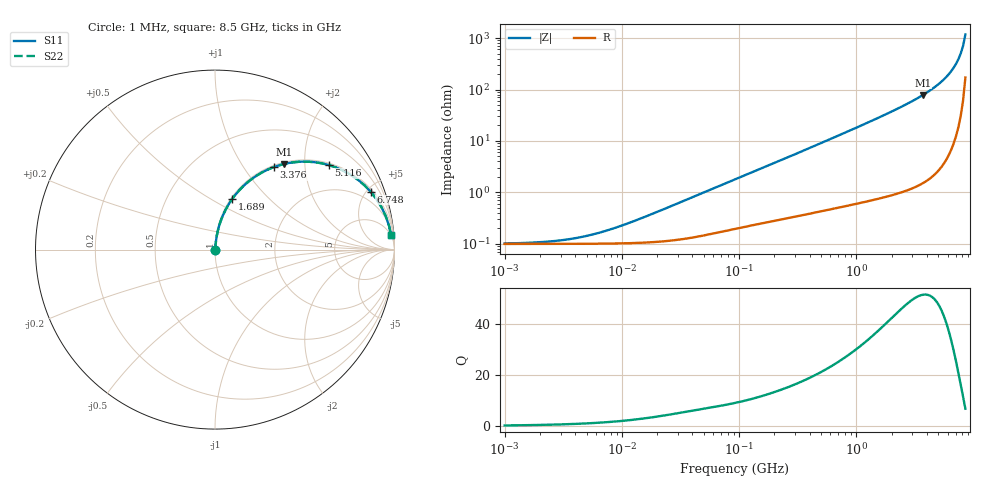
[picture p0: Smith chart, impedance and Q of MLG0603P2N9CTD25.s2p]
! S-Parameter Data Generated by TDK Corporation
! Copyright(C) 2025 TDK Corporation.
! All Rights Reserved.
! TDK P/N: MLG0603P2N9CTD25 (SMD / SMT Inductor (Coil))
! Property: L=2.9nH at 500MHz
! Size(LxWxT): 0.6x0.3x0.3mm
! Model Type: s2p (Touchstone File Format Version 1.0)
! Frequency: DC=Yes Start=1MHz Stop=8500MHz 198points Log-sweep
! Model Generated on Feb. 6, 2025
! Terms and conditions regarding TDK Simulation Models:
! 1)This simulation model is being provided solely for informational
!  purposes. Please refer to the specifications of the products in
!  terms of detailed characteristics of such products.
! 2)In no event shall TDK Corporation of any of its subsidiaries be
!  liable for any loss or damage arising, directly or indirectly,
!  from any information contained in this simulation model, including,
!  but not limited to loss or damages arising from any inaccuracies,
!  omissions or errors in connection with such information.
! 3)Any and all copyrights on this simulation model are owned by
!  TDK Corporation.  Duplication or redistribution of this simulation
!  model without prior written permission from TDK Corporation
!  is prohibited.
! 4)This simulation model is subject to any modification or change
!  without any prior notice.
! 5)Neither TDK Corporation nor any of its subsidiaries shall make any
!  warranty, express or implied, including but not limited to the
!  correctness, implied warranties of merchantability and fitness for
!  a particular purpose with respect to this simulation models.
! 6)The use of this simulation model shall be deemed to have consented
!  to the terms and conditions hereof.
! Port Assignments:
!  1 ---@@@--- 2
! Applicable Conditions:
!  Temperature = 25 degC
!  DC Bias Current = 0 A
!  Small Signal Operation
# Hz S MA R 50
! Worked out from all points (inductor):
!   197 points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, 1 MHz to 8.5 GHz, reference 50 ohm
!   read as one part in series: L = 3.22 nH near 15.95 MHz
!   highest Q = 51.5 at 3.703 GHz (marker M1), where L = 3.37 nH
!   S11 on the Smith chart (normalised r, x): 1 MHz: 1.00, +0.00; 1.689 GHz: 1.02, +0.62; 3.376 GHz: 1.03, +1.39; 5.116 GHz: 1.06, +2.64; 6.748 GHz: 1.18, +5.29; 8.5 GHz: 4, +23
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1000000  0.00102 11.5  0.999 -0.0  0.999 -0.0  0.00102 11.5
2403882  0.001114 26.0  0.999 -0.0  0.999 -0.0  0.001114 26.0
4587603  0.001371 42.8  0.999 -0.1  0.999 -0.1  0.001371 42.8
8755050  0.00205 60.1  0.999 -0.1  0.999 -0.1  0.00205 60.1
2.10461e7  0.004394 75.2  0.9989 -0.2  0.9989 -0.2  0.004394 75.2
9.219544e7  0.01781 82.7  0.9979 -1.0  0.9979 -1.0  0.01781 82.7
2.116287e8  0.03935 83.6  0.9964 -2.2  0.9964 -2.2  0.03935 83.6
4.229561e8  0.07688 82.7  0.9931 -4.4  0.9931 -4.4  0.07688 82.7
8.852465e8  0.1578 78.9  0.9819 -9.1  0.9819 -9.1  0.1578 78.9
1.689417e9  0.2954 71.4  0.9479 -17.2  0.9479 -17.2  0.2954 71.4
1.940355e9  0.3374 68.9  0.9333 -19.7  0.9333 -19.7  0.3374 68.9
2.559585e9  0.4385 62.8  0.8894 -26.0  0.8894 -26.0  0.4385 62.8
3.37643e9  0.5645 54.5  0.8145 -34.4  0.8145 -34.4  0.5645 54.5
3.703002e9  0.6118 51.2  0.7793 -37.7  0.7793 -37.7  0.6118 51.2
4.453958e9  0.7122 43.5  0.688 -45.4  0.688 -45.4  0.7122 43.5
5.115526e9  0.7893 36.7  0.5975 -52.1  0.5975 -52.1  0.7893 36.7
5.87536e9  0.8626 29.0  0.4849 -59.6  0.4849 -59.6  0.8626 29.0
6.748056e9  0.9252 20.4  0.3496 -67.6  0.3496 -67.6  0.9252 20.4
7.400733e9  0.957 14.3  0.248 -72.9  0.248 -72.9  0.957 14.3
7.750377e9  0.9691 11.2  0.1944 -75.3  0.1944 -75.3  0.9691 11.2
8.116539e9  0.9783 8.0  0.1396 -77.1  0.1396 -77.1  0.9783 8.0
8.5e9  0.9843 4.8  0.08387 -76.9  0.08387 -76.9  0.9843 4.8
